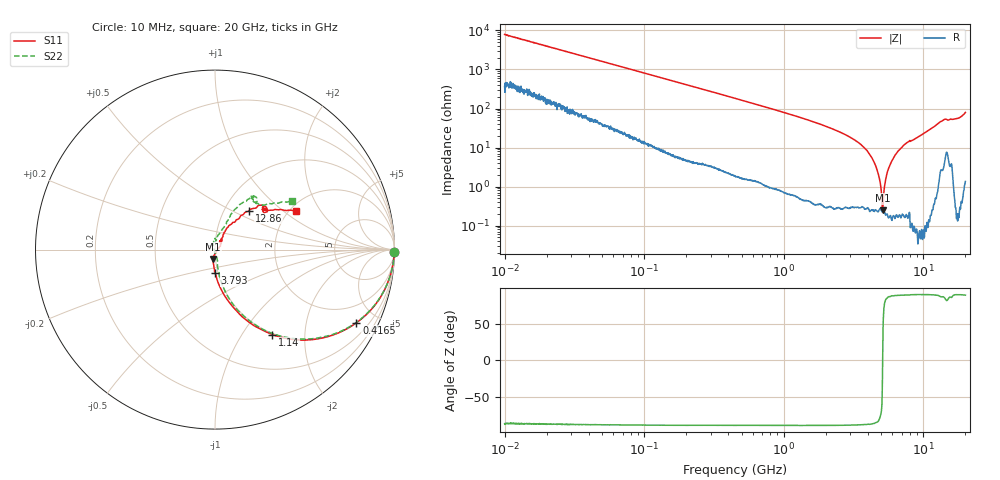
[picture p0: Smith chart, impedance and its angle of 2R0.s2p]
!Keysight Technologies,P5008B,MY61100088,A.16.20.02
!Date: Friday, August 30, 2024 11:11:16
!Correction: S11(C  2-Port  )
!S21(C  2-Port  )
!S12(C  2-Port  )
!S22(C  2-Port  )
!S2P File: Measurements: S11, S21, S12, S22:Log Frequency Sweep
# Hz S  dB  R 50
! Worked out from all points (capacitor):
!   1601 points, 10 MHz to 20 GHz, reference 50 ohm
!   read as one part in series: C = 2.02 pF near 10.39 MHz
!   lowest |Z| = 250 mohm at 5.116 GHz (marker M1)
!   series resonance near 5.107 GHz, so ESL is about 480 pH
!   S11 on the Smith chart (normalised r, x): 10 MHz: open; 416.5 MHz: 1.01, -3.86; 1.14 GHz: 0.98, -1.38; 3.793 GHz: 0.96, -0.26; 12.86 GHz: 1.30, +0.62; 20 GHz: 2.17, +1.24
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1e7  -0.00 -0.7  -37.92 86.6  -37.92 86.5  -0.01 -0.7
3.555162e7  -0.02 -2.6  -27.06 85.7  -27.06 85.7  -0.02 -2.6
1.263918e8  -0.13 -9.0  -16.31 80.3  -16.31 80.3  -0.12 -8.9
4.164548e8  -1.04 -27.4  -6.91 62.2  -6.91 62.2  -1.04 -27.1
4.472136e8  -1.18 -29.1  -6.42 60.5  -6.43 60.5  -1.18 -28.8
1.14013e9  -4.86 -56.0  -1.77 33.9  -1.77 33.9  -4.86 -55.3
1.589917e9  -7.28 -65.8  -0.93 24.3  -0.94 24.3  -7.27 -64.7
2.693912e9  -12.40 -80.0  -0.28 11.2  -0.28 11.1  -12.37 -76.3
3.792536e9  -17.71 -90.6  -0.10 3.6  -0.10 3.6  -17.61 -79.8
5.115731e9  -25.37 -101.7  -0.03 -3.1  -0.03 -3.1  -25.28 -77.6
5.652411e9  -29.29 -100.4  -0.01 -5.3  -0.01 -5.4  -29.70 -81.1
5.927413e9  -32.28 -93.2  -0.00 -6.4  -0.01 -6.5  -33.21 -86.2
6.245393e9  -38.33 -55.2  0.00 -7.6  0.00 -7.6  -43.49 -112.9
6.395515e9  -37.92 -21.9  0.00 -8.2  0.00 -8.2  -47.41 175.9
6.518206e9  -36.78 5.0  0.00 -8.6  0.00 -8.7  -41.17 129.1
6.933443e9  -30.89 31.3  0.01 -10.1  0.00 -10.2  -32.09 112.4
7.445538e9  -26.59 45.4  -0.00 -11.9  0.00 -12.0  -27.16 100.1
8.709232e9  -24.93 60.8  0.01 -16.1  0.00 -16.2  -24.95 80.3
1.285753e10  -10.82 48.9  -0.40 -31.7  -0.41 -31.8  -10.86 61.2
1.413906e10  -8.69 41.4  -0.85 -35.8  -0.85 -35.9  -8.67 53.6
1.717946e10  -9.03 40.6  -0.55 -42.6  -0.55 -42.7  -9.05 52.9
2e10  -6.02 25.2  -1.34 -59.7  -1.35 -59.8  -5.92 32.4
